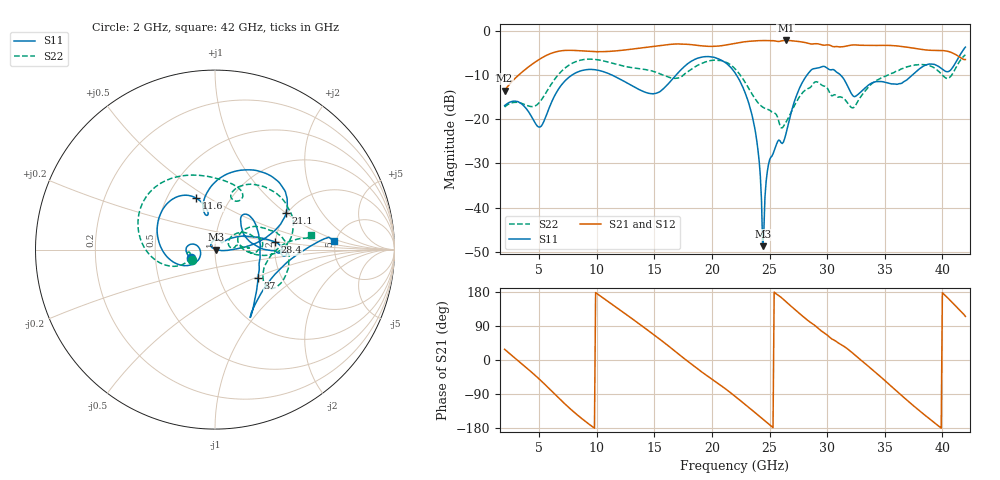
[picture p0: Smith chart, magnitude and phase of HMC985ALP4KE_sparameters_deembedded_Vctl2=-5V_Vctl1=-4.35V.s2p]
!s2p File: Measurements: S11, S21, S12, S22
# GHz S dB R 50.0
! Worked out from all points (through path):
!   401 points, 2 GHz to 42 GHz, reference 50 ohm
!   highest |S21| = -2.06 dB at 26.4 GHz (marker M1); lowest = -13.4 dB at 2 GHz (marker M2)
!   lowest |S11| = -48.8 dB at 24.4 GHz (marker M3), VSWR 1.01, Z = 50.4 + j0.0337 ohm
!   |S11| at or under -10 dB: start of sweep to 7.805 GHz; 22.14 GHz to 28.23 GHz (6.086 GHz wide, 24.2 % of centre); 31.19 GHz to 37.36 GHz (6.169 GHz wide, 18 % of centre)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
!   |S22| runs from -21.9 to -5.3 dB; largest |S21 - S12| = 0.001
!   S11 on the Smith chart (normalised r, x): 2 GHz: 0.76, -0.07; 11.6 GHz: 0.69, +0.44; 21.1 GHz: 1.97, +1.02; 28.4 GHz: 2.00, +0.19; 37 GHz: 1.52, -0.53; 42 GHz: 4.77, +0.83
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2  -16.86 -161.8  -13.44 28.2  -13.44 28.2  -17.16 -155.7
5  -21.75 -172.6  -6.38 -50.1  -6.38 -50.1  -16.18 -159.9
6.3  -14.83 -150.5  -4.76 -88.3  -4.76 -88.3  -11.04 -161.6
8.7  -8.90 150.3  -4.44 -154.6  -4.44 -154.6  -6.47 151.3
11.6  -10.28 110.3  -4.45 141.0  -4.45 141.0  -7.40 103.5
13.6  -13.11 101.1  -3.85 97.2  -3.85 97.2  -8.44 75.9
15.4  -13.80 105.7  -3.25 56.4  -3.25 56.4  -9.53 62.4
17.9  -7.32 80.1  -2.95 -3.6  -2.94 -3.5  -9.16 72.3
21.1  -6.99 27.4  -3.14 -74.4  -3.14 -74.4  -6.87 16.1
22  -9.40 16.8  -2.71 -95.6  -2.71 -95.6  -8.48 0.7
23.6  -20.46 -0.2  -2.18 -135.4  -2.17 -135.3  -14.74 -3.9
24  -27.09 -7.3  -2.11 -145.4  -2.11 -145.4  -16.22 1.7
24.4  -48.78 5.3  -2.08 -155.5  -2.08 -155.5  -17.18 7.4
25  -29.20 133.3  -2.11 -170.8  -2.11 -170.7  -17.88 11.0
26.4  -23.50 42.8  -2.06 154.5  -2.06 154.6  -20.75 33.1
28.4  -9.41 7.2  -2.73 102.6  -2.73 102.6  -12.92 18.4
28.7  -8.60 2.1  -2.87 96.4  -2.87 96.4  -12.21 16.6
32.5  -14.68 33.2  -3.08 10.6  -3.08 10.7  -16.63 28.7
35.4  -11.78 19.0  -3.19 -64.8  -3.19 -64.7  -9.79 19.5
37  -10.83 -33.5  -3.62 -107.9  -3.62 -107.8  -8.02 5.1
39.8  -8.18 -56.8  -4.33 -177.3  -4.33 -177.3  -9.37 -34.9
42  -3.58 4.2  -6.40 115.1  -6.40 115.1  -5.31 8.9
